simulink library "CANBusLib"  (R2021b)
settings: Solver=VariableStepAuto  StartTime=0.0  StopTime=10.0  RelTol=1e-3
undefined symbols (not defined in the file or in its folder): Endian, Little

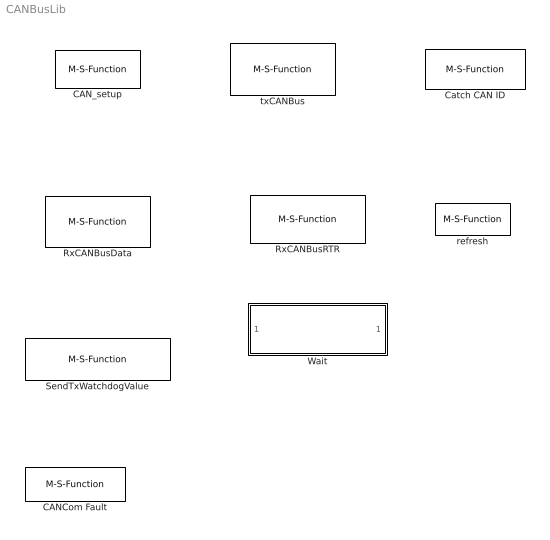
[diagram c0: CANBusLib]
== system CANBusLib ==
  CANCom Fault : M-S-Function  FunctionName=CAN_ComFault2  Parameters=g1_cmbObjectID  mask(CAN bus communication diagnosis based on RxWatchdog){g1_cmbObjectID=0}
      mask prompts: g1_cmbObjectID "Object ID for multiple CAN bus controllers:"
      mask help: This is based on RxWatchdog's CAN bus communication fault diagnosis block. It will output true when RxWatchdog thinks CAN Bus communication has problem. You must enable RxWtachdog, otherwise, you cannot get fault output.
  CAN_setup : M-S-Function  Priority=1  FunctionName=CAN_setup2  Parameters=g1_cmbPortName, g2_cmbBaudRate,g3_chkEcho,g59_chkTerminator,g4_cmbObjectID,g5_chkEnableSync,g6_rdoSyncSource,g7_ediSyncCANID,g8_chkSyncExtended,g9_ediSyncPeriod,g10_chkRxWDEnable,g11_cmbRxWDDLC,g55_chkRxWDCANID,g56_chkRxWDExtended,g12_cmbRxWDLen,g13_cmbRxWDStartPos,g14_ediRxWDPeriod,g_60_cmbRxWDMode,g15_chkTxWDEnable,g16_cmbTxWDDLC,g57_chkTxWDCANID,g58_chkTxWDExtended,g17_cmbTxWDLen,g18_cmbTxWDSta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  mask(CAN Bus controller setup){g1_cmbPortName="COM17", g2_cmbBaudRate=250000, g3_chkEcho=off, g59_chkTerminator=on, g4_cmbObjectID=0, g5_chkEnableSync=off, g6_rdoSyncSource=Sync by dedicated Receiving frame, g7_ediSyncCANID=[], g8_chkSyncExtended=off, g9_ediSyncPeriod=[], g10_chkRxWDEnable=off, g11_cmbRxWDDLC=1, g55_chkRxWDCANID=[], g56_chkRxWDExtended=off, g12_cmbRxWDLen=1, g13_cmbRxWDStartPos=1, g14_ediRxWDPeriod=[], g_60_cmbRxWDMode=0, g15_chkTxWDEnable=off, g16_cmbTxWDDLC=1, g57_chkTxWDCANID=[], g58_chkTxWDExtended=off, g17_cmbTxWDLen=1, g18_cmbTxWDStartPos=1, g19_ediTxWDPeriod=[], g_61_cmbTxWDMode=0, g20_ediF1=0, g21_chkExt4F1=off, g22_ediF2=0, g23_chkExt4F2=off, g24_ediF3=0, g25_chkExt4F3=off, g26_ediF4=0, g27_chkExt4F4=off, g28_ediF5=0, g29_chkExt4F5=off, g30_ediF6=0, g31_chkExt4F6=off, g32_ediF7=0, g33_chkExt4F7=off, g34_ediF8=0, g35_chkExt4F8=off, g36_ediM1=0, g37_ediF9=0, g38_chkExt4F9=on, g39_ediF10=0, g40_chkExt4F10=on, g41_ediF11=0, g42_chkExt4F11=on, g43_ediF12=0, g44_chkExt4F12=on, g45_ediM2=0, g46_ediF13=0, g47_chkExt4F13=off, g48_ediF14=0, g49_chkExt4F14=on, g50_ediF15=0, g51_chkExt4F15=on, g52_ediF16=0, g53_chkExt4F16=on, g54_ediM3=0, g62_autoFresh=on}
      mask prompts: g1_cmbPortName "Connect to:"; g2_cmbBaudRate "CAN Bus Baud Rate:"; g3_chkEcho "Echo On"; g59_chkTerminator "Enable 120 Ω terminator"; g4_cmbObjectID "Object ID for multiple CAN bus controllers:"; g5_chkEnableSync "Enable Sync:"; g6_rdoSyncSource "Sync Source Selection"; g7_ediSyncCANID "SyncCAN ID:"; g8_chkSyncExtended "Sync uses extended CAN ID"; g9_ediSyncPeriod "Sync periods in ms:"; g10_chkRxWDEnable "Rx Watchdog Enable"; g11_cmbRxWDDLC "Rx Watchdog Frame DLC"; g55_chkRxWDCANID "RxWatchdogCAN ID:"; g56_chkRxWDExtended "RxWatchdog uses extended ID"; g12_cmbRxWDLen "RxWatchdog Counter byte qty"; g13_cmbRxWDStartPos "RxWatchdog Start position:"; g14_ediRxWDPeriod "RxWatchdog Periods:"; g_60_cmbRxWDMode "RxWatchdog Mode"; g15_chkTxWDEnable "TxWatchdog Enable"; g16_cmbTxWDDLC "Tx Watchdog Frame DLC"; g57_chkTxWDCANID "TxWatchdogCAN ID:"; g58_chkTxWDExtended "TxWatchdog uses extended ID"; g17_cmbTxWDLen "TxWatchdog Counter byte qty"; g18_cmbTxWDStartPos "TxWatchdog Start position:"; g19_ediTxWDPeriod "TxWatchdog Periods:"; g_61_cmbTxWDMode "TxWatchdog Mode"; g20_ediF1 "Filter1"; g21_chkExt4F1 "Extended"; g22_ediF2 "Filter2"; g23_chkExt4F2 "Extended"; g24_ediF3 "Filter3"; g25_chkExt4F3 "Extended"; g26_ediF4 "Filter4"; g27_chkExt4F4 "Extended"; g28_ediF5 "Filter5"; g29_chkExt4F5 "Extended"; g30_ediF6 "Filter6"; g31_chkExt4F6 "Extended"; g32_ediF7 "Filter7"; g33_chkExt4F7 "Extended"; g34_ediF8 "Filter8"; g35_chkExt4F8 "Extended"; g36_ediM1 "Mask1"; g37_ediF9 "Filter9"; g38_chkExt4F9 "Extended"; g39_ediF10 "Filter10"; g40_chkExt4F10 "Extended"; g41_ediF11 "Filter11"; g42_chkExt4F11 "Extended"; g43_ediF12 "Filter12"; g44_chkExt4F12 "Extended"; g45_ediM2 "Mask2"; g46_ediF13 "Filter13"; g47_chkExt4F13 "Extended"; g48_ediF14 "Filter14"; g49_chkExt4F14 "Extended"; g50_ediF15 "Filter15"; g51_chkExt4F15 "Extended"; g52_ediF16 "Filter16"; g53_chkExt4F16 "Extended"; g54_ediM3 "Mask3"; g62_autoFresh "Enable auto-fresh"
      mask help: It sets up CAN Bus controller.. You must firstly set up CAN Bus controller before you use any CAN bus controller block. Parameter "Object ID for multilple CAN bus controllers" is for CAN bus controller object ID. We could use multiple CAN bus controllers, so we use this parameter to identify which CAN bus controller is used for CAN Bus controller operation blocks.
      mask init:
      | %set_param('CANBusLib','Lock','off');
      | set_param(gcs,'Lock','off');
      | set_param(gcbh, "MaskSelfModifiable",'on');
  Catch CAN ID : M-S-Function  FunctionName=catchCANID2  Parameters="g1_ObjectID, g2_CANID,  g3_Extended,g4_chkCatchLast,g5_lastFrameNo"  mask(Catch your interesting CAN ID or Catch the last frame in long data frames){g1_ObjectID=0, g2_CANID=0, g3_Extended=off, g4_chkCatchLast=on, g5_lastFrameNo=2}
      mask prompts: g1_ObjectID "Object ID for multiple CAN bus controllers:"; g2_CANID "Catch CAN ID:"; g3_Extended "Extended"; g4_chkCatchLast "Catch last frame only"; g5_lastFrameNo "The last frame number:"
      mask help: It will set Outport "Got' to true for one "Pulse" when your interesting CAN ID caught.
  RxCANBusData : M-S-Function  FunctionName=rxCANBusData2  Parameters=g1_ObjectID, g2_CANID, g3_Extended,g4_Datatype, g5_Endian, g6_Longframe, g7_OutDataQTY,g8_FirstFrameNo  mask(Receive CAN Bus Data){g1_ObjectID=0, g2_CANID=479, g3_Extended=off, g4_Datatype=[ "uint16", "uint8"], g5_Endian=Little-Endian, g6_Longframe=off, g7_OutDataQTY=8, g8_FirstFrameNo=0}
      mask prompts: g1_ObjectID "Object ID for multiple CAN bus controllers:"; g2_CANID "Received CAN ID:"; g3_Extended "Extended"; g4_Datatype "Data Type (Such as "uint8", ... , "int64" , "single","double")"; g5_Endian "Endian for multiple bytes data type:"; g6_Longframe "Long Frames"; g7_OutDataQTY "Output Data item Qty:"; g8_FirstFrameNo "The 1st frame Number:"
      mask help: Receive CAN Bus Data frame. This is non-block function. If no any data frame received for your interesting CAN ID, Outport Rx will be false
  RxCANBusRTR : M-S-Function  FunctionName=rxCANBusRTR2  Parameters="g1_ObjectID, g2_CANID,  g3_Extended"  mask(Receive RTR frame){g1_ObjectID=0, g2_CANID=0, g3_Extended=off}
      mask prompts: g1_ObjectID "Object ID for multiple CAN bus controllers:"; g2_CANID "Received CAN ID:"; g3_Extended "Extended"
      mask help: Receive CAN Bus Remote Request frame. This is non-block function. If no any RTR frame received for your interesting CAN ID, Outport Rx will be false
  SendTxWatchdogValue : M-S-Function  FunctionName=sendTxWatchdogValue2  Parameters=g1_cmbObjectID  mask(send TxWatchdog counter Value){g1_cmbObjectID=0}
      mask prompts: g1_cmbObjectID "Object ID for multiple CAN bus controllers:"
      mask help: send TxWatchdog counter Value. It is only used in TxWatchdog mode 0. For other modes, it is no use.
  Wait : MATLAB Function  TreatAsAtomicUnit=on  mask(wait block){Waitms=500}
      mask prompts: Waitms "Time in ms for waiting:"
      mask help: This is for waiting in ms when Inport EnIn=true or greater than 0. Min=50ms. However Windows OS is not realtime OS, It cannot guarantee. Max = max number of 32 bits of unsigned integer. Outport EnOut=true if Inport EnIn=true or greater than 0 Outport EnOut=false if Inport EnIn=false or Not greater than 0. This waiting time is real time, not simulated time. This function is block function.
  refresh : M-S-Function  FunctionName=refresh2  Parameters=g1_cmbObjectID  mask(refresh CAN Bus receiver buffer){g1_cmbObjectID=0}
      mask prompts: g1_cmbObjectID "Object ID for multiple CAN bus controllers:"
      mask help: When input port "En" >0 or true, it will refresh CAN bus receiver frames buffers
  txCANBus : M-S-Function  FunctionName=txCANBus2  Parameters=g1_cmbObjectID, g2_CANID,g3_Extended,g4_RTR,g5_Datatype,g6_Endian,g7_Longframe,g8_FirstFrameNo,g9_LastFrameDLC8  mask(Transmit CAN BUS Data/RTR frames.){g1_cmbObjectID=0, g2_CANID=0, g3_Extended=off, g4_RTR=off, g5_Datatype=["uint8", "uint16"], g6_Endian=Little-Endian, g7_Longframe=off, g8_FirstFrameNo=1, g9_LastFrameDLC8=on}
      mask prompts: g1_cmbObjectID "Object ID for multiple CAN bus controllers:"; g2_CANID "Transmitted CAN ID:"; g3_Extended "Extended"; g4_RTR "Remote Request Frame"; g5_Datatype "Data Type (Such as "uint8", ... , "int64" , "single","double")"; g6_Endian "Endian for multiple bytes data type:"; g7_Longframe "Long Frames"; g8_FirstFrameNo "The 1st frame Number:"; g9_LastFrameDLC8 "The last frame DLC keeps 8"
      mask help: Transmit CAN bus single Data/RTR frame. Or transmit multiple Data frames.

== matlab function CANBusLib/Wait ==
function out=fcn(in, Waitms)
    if in==true
        pause(Waitms/1000.0);
        out=true;  % Delay done
    elseif in>0
        pause(Waitms/1000.0);
        out=true;  % Delay done
    else
        out=false;  % No dealy
        return;
    end
